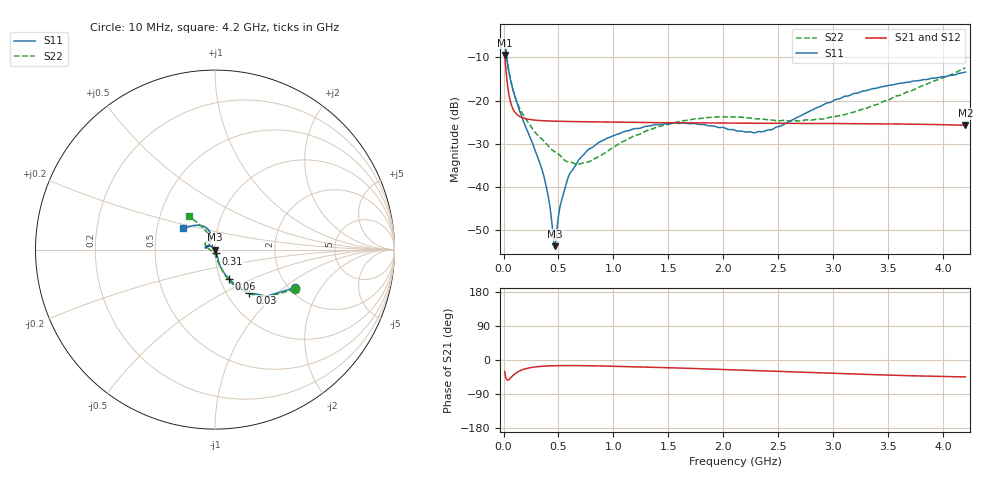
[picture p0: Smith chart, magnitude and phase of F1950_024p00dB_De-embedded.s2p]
! Integrated Device Technology
! Corporate Headquarters
! 6024 Silver Creek Valley Road
! San Jose, CA 95138  USA
! Phone:  1-408-284-8200
! Toll Free:  1-800-223-1366
! Webpage:  http://www.idt.com/
! Timing and RF Division
! 515 Groton Road, Suite 102
! Westford, MA 01886-6024
! Device:  F1950
! Description: 7-bit 0.25 dB Digital Step Attenuator
! Frequency:  150.0 -  4000.00 MHz
! Package:  4x4 mm Thin QFN Plastic Package: 24 pin
! Ports:  2 RF, 12 DC
!  Pin  1  = D0
!  Pin  2  = VDD
!  Pin  3  = Vmode
!  Pin  4  = GND
!  Pin  5  = RF1  =  Port 1
!  Pin  6  = GND
!  Pin  7  = GND
!  Pin  8  = GND
!  Pin  9  = GND
!  Pin 10  = GND
!  Pin 11  = GND
!  Pin 12  = GND
!  Pin 13  = GND
!  Pin 14  = RF2  =  Port 2
!  Pin 15  = GND
!  Pin 16  = LE
!  Pin 17  = CLK
!  Pin 18  = DATE
!  Pin 19  = D6
!  Pin 20  = D5
!  Pin 21  = D4
!  Pin 22  = D3
!  Pin 23  = D2
!  Pin 24  = D1
! State:  96
! Atten State:  24.00 dB
! Voltage:  +5.00 Volts
! Current:  Not Measured mA
! Data:  The device was measured on a the F195X evaluation board which has
!  individual transmission lines to the RF pins.  Data was collected
!  using a calibrated network analyzer.  The evaluation board was
!  de-embedded using a TRL calibration technique.
!  The reference plane is the edge of the package pin.
! Misc:  Board 2019
!  Action Tracker AT0250
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# GHz S dB R 50
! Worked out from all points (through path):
!   420 points, 10 MHz to 4.2 GHz, reference 50 ohm
!   highest |S21| = -9.42 dB at 10 MHz (marker M1); lowest = -25.7 dB at 4.2 GHz (marker M2)
!   group delay of S21, straight-line fit = 18.5 ps
!   lowest |S11| = -53.7 dB at 470 MHz (marker M3), VSWR 1.00, Z = 49.8 - j0.0441 ohm
!   |S11| at or under -10 dB: 28.74 MHz to end of sweep
!   |S22| runs from -34.8 to -6.1 dB; largest |S21 - S12| = 0.00011
!   S11 on the Smith chart (normalised r, x): 10 MHz: 2.14, -1.20; 30 MHz: 1.28, -0.67; 60 MHz: 1.10, -0.37; 310 MHz: 1.01, -0.04; 4.2 GHz: 0.68, +0.17
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0.01  -6.14 -25.5  -9.42 -30.4  -9.42 -30.3  -6.08 -26.5
0.03  -10.25 -51.3  -14.96 -52.2  -14.96 -52.2  -10.20 -52.7
0.06  -14.80 -64.3  -19.97 -48.6  -19.97 -48.6  -14.59 -65.8
0.09  -17.86 -69.8  -22.14 -39.9  -22.14 -39.9  -17.82 -70.2
0.14  -21.88 -72.5  -23.56 -29.7  -23.56 -29.7  -21.42 -74.6
0.31  -33.06 -72.6  -24.59 -17.6  -24.58 -17.6  -28.00 -83.6
0.39  -40.11 -73.6  -24.70 -15.9  -24.70 -15.9  -30.01 -87.2
0.42  -44.19 -82.7  -24.73 -15.5  -24.73 -15.5  -30.85 -89.4
0.45  -50.97 -108.1  -24.76 -15.2  -24.76 -15.2  -31.59 -93.8
0.47  -53.71 -167.6  -24.77 -15.1  -24.77 -15.1  -31.91 -97.1
0.52  -43.89 145.9  -24.81 -14.8  -24.80 -14.8  -32.84 -101.8
0.58  -38.40 137.9  -24.84 -14.7  -24.84 -14.7  -34.15 -113.6
0.71  -33.01 139.6  -24.89 -14.9  -24.89 -14.9  -34.52 -138.2
0.99  -28.21 148.5  -25.00 -16.4  -24.99 -16.4  -30.98 -178.4
1.41  -25.55 164.0  -25.11 -19.7  -25.10 -19.7  -26.04 161.7
1.73  -25.30 169.5  -25.16 -22.4  -25.16 -22.4  -24.26 153.3
2.11  -26.94 159.7  -25.22 -26.2  -25.22 -26.2  -23.86 143.5
2.43  -26.80 128.4  -25.25 -29.1  -25.25 -29.1  -24.46 133.1
2.81  -22.17 106.6  -25.29 -33.1  -25.29 -33.1  -24.50 117.9
3.19  -18.34 109.6  -25.34 -37.0  -25.34 -37.0  -22.65 112.1
3.51  -16.45 118.3  -25.39 -39.9  -25.39 -39.9  -19.76 114.5
4.2  -13.41 146.2  -25.71 -44.5  -25.71 -44.6  -12.44 127.8
